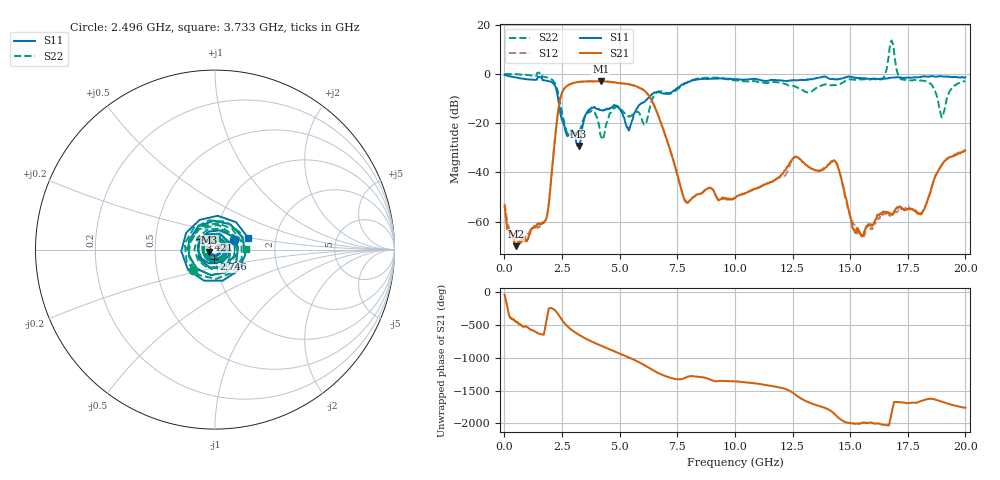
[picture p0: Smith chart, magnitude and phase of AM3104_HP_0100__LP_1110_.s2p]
!Created with skrf (http://scikit-rf.org).
# Hz S RI R 50.0
!freq ReS11 ImS11 ReS21 ImS21 ReS12 ImS12 ReS22 ImS22
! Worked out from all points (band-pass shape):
!   1601 points, 10 MHz to 20 GHz, reference 50 ohm
!   highest |S21| = -2.90 dB at 4.183 GHz (marker M1); lowest = -70.0 dB at 509.8 MHz (marker M2)
!   |S21| within 3 dB of the highest: 2.602 GHz to 5.924 GHz (3.323 GHz wide, 77.9 % of centre)
!   lowest |S11| = -29.3 dB at 3.221 GHz (marker M3), VSWR 1.07, Z = 46.9 - j1.17 ohm
!   |S11| at or under -10 dB: 2.329 GHz to 6.217 GHz (3.888 GHz wide, 91 % of centre)
!   |S22| runs from -26.7 to 13.6 dB; largest |S21 - S12| = 0.077
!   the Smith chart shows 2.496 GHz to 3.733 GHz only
!   S11 on the Smith chart (normalised r, x): 2.496 GHz: 1.23, +0.13; 2.746 GHz: 0.98, -0.11; 3.421 GHz: 0.84, +0.10; 3.733 GHz: 1.44, +0.20
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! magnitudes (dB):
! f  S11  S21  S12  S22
! 10 MHz  -0.4  -53.8  -52.7  0.0
! 509.8 MHz  -1.4  -70.0  -66.9  -0.1
! 1.809 GHz  -2.7  -59.0  -59.2  -1.3
! 2.496 GHz  -18.6  -7.7  -7.7  -15.5
! 2.746 GHz  -25.2  -4.7  -4.7  -24.2
! 3.221 GHz  -29.3  -3.2  -3.3  -24.4
! 3.346 GHz  -23.7  -3.1  -3.2  -21.0
! 3.421 GHz  -19.8  -3.1  -3.1  -18.6
! 3.733 GHz  -14.2  -3.0  -3.0  -15.3
! 4.183 GHz  -14.7  -2.9  -2.9  -25.2
! 5.395 GHz  -23.0  -4.2  -4.2  -17.4
! 6.107 GHz  -11.0  -7.1  -7.1  -20.6
! 6.682 GHz  -7.3  -17.0  -17.0  -7.1
! 7.869 GHz  -3.7  -51.9  -51.4  -3.7
! 10.01 GHz  -2.2  -50.4  -50.3  -2.7
! 13.34 GHz  -2.2  -38.6  -38.6  -7.0
! 14.38 GHz  -2.1  -35.8  -36.1  -4.5
! 15.39 GHz  -1.7  -64.3  -65.3  -2.2
! 16.68 GHz  -1.7  -56.5  -57.2  7.3
! 18.09 GHz  -1.0  -56.6  -56.8  -2.7
! 18.98 GHz  -1.0  -36.9  -36.8  -17.6
! 20 GHz  -1.3  -31.1  -30.8  -2.9
